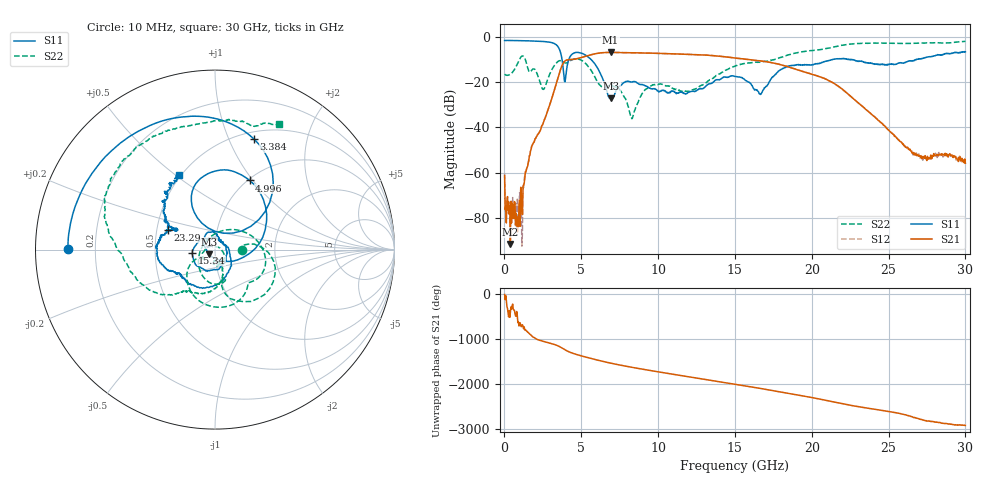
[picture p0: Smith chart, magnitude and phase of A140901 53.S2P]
!  2-Port S-parameters saved by WinCal
! VAR MeasName=S-Parameters (CALIBRATED_DATA) read from VNA (N5244A)
! VAR MeasDate=11/3/2014 9:36:04 AM
! VAR NAME=A140901 53
! VAR FILENAME=A140901 53.S2P
! VAR DATE=11/3/2014 9:36:04 AM
! VAR PHYS_PORTS=1,2
# Hz S RI R 50
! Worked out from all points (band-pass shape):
!   801 points, 10 MHz to 30 GHz, reference 50 ohm
!   highest |S21| = -6.95 dB at 6.908 GHz (marker M1); lowest = -91.4 dB at 384.9 MHz (marker M2)
!   |S21| within 3 dB of the highest: 4.578 GHz to 15.69 GHz (11.12 GHz wide, 110 % of centre)
!   lowest |S11| = -27.2 dB at 6.945 GHz (marker M3), VSWR 1.09, Z = 46.6 - j2.54 ohm
!   |S11| at or under -10 dB: 3.744 GHz to 4.194 GHz (449.6 MHz wide, 11.3 % of centre); 5.619 GHz to 21.45 GHz (15.83 GHz wide, 117 % of centre); 22.4 GHz to 26.84 GHz (4.441 GHz wide, 18 % of centre)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
!   |S22| runs from -36.2 to -2.1 dB; largest |S21 - S12| = 0.0033
!   S11 on the Smith chart (normalised r, x): 10 MHz: 0.10, +0.00; 3.384 GHz: 0.58, +1.24; 4.996 GHz: 1.02, +0.96; 15.34 GHz: 0.77, -0.03; 23.29 GHz: 0.57, +0.14; 30 GHz: 0.49, +0.52
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1e7  -0.8185 0.00212  0.000848 -0.000159  -0.000215 0.000942  0.1478 -0.00114
3.84875e8  -0.8092 0.1253  2.13e-05 -1.67e-05  9.98e-06 -7.83e-05  0.1473 0.0138
8.722125e8  -0.7638 0.2791  1.4e-05 0.000106  1.57e-05 4.74e-05  0.2622 0.011
1.734425e9  -0.6015 0.5269  -0.00314 0.000952  -0.0032 0.00105  0.0586 -0.1623
2.521662e9  -0.3316 0.7039  0.0112 0.00566  0.0112 0.00569  -0.0553 0.0408
3.383875e9  0.2183 0.615  0.0476 -0.0819  0.0474 -0.0818  0.2632 0.00758
3.946188e9  0.0016 0.1012  -0.278 -0.0859  -0.2777 -0.086  0.1878 -0.1829
4.995838e9  0.1929 0.3855  0.1519 0.3092  0.1514 0.3088  -0.0774 -0.2924
5.033325e9  0.2062 0.3738  0.1723 0.3018  0.1717 0.3016  -0.0893 -0.2845
5.895538e9  0.2452 0.0314  0.398 -0.1252  0.3983 -0.1241  -0.1127 -0.0576
6.9077e9  -0.0295 -0.033  -0.0707 -0.4435  -0.0699 -0.4433  -0.0645 -0.0549
6.945188e9  -0.0342 -0.0272  -0.0918 -0.4393  -0.0913 -0.439  -0.0653 -0.0545
8.294738e9  -0.0183 0.0981  -0.4309 0.0888  -0.4302 0.0882  0.00141 0.0154
1.001916e10  0.0166 0.0601  0.1709 0.3918  0.1703 0.3911  0.0155 -0.087
1.268078e10  0.0678 -0.0172  0.0642 -0.3902  0.0641 -0.3899  0.0246 -0.075
1.5005e10  -0.1168 -0.0628  -0.2928 0.1673  -0.2913 0.1683  -0.00809 -0.224
1.534239e10  -0.127 -0.0167  -0.2181 0.2438  -0.2181 0.2435  -0.041 -0.2373
1.74042e10  0.0904 -0.0862  0.2581 0.0607  0.2582 0.0623  -0.1882 -0.2362
2.002832e10  -0.1989 -0.132  -0.1232 -0.0803  -0.123 -0.0814  -0.4805 -0.1001
2.328974e10  -0.2613 0.1108  0.0291 -0.00147  0.0294 -0.00128  -0.5284 0.4775
2.501416e10  -0.2109 0.1136  -0.00107 -0.00865  -0.000853 -0.00865  -0.2618 0.6653
3e10  -0.1979 0.4165  0.00111 -0.00119  0.00112 -0.00103  0.3589 0.6977
